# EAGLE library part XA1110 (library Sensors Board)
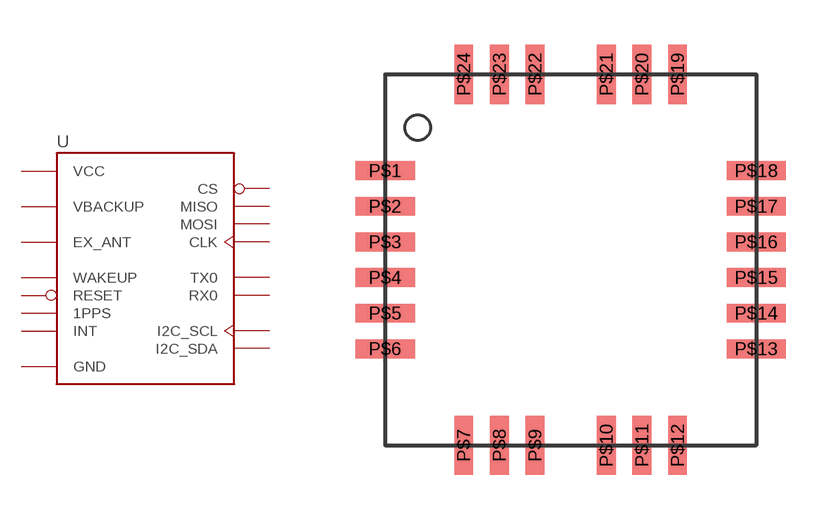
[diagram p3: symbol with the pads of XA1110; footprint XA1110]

Designator prefix -

## XA1110  [XA1110]
P$1  GND  sup
P$2  EX_ANT  in
P$3  GND  sup
P$4  GND  sup
P$5  GND  sup
P$6  GND  sup
P$7  VCC  sup
P$8  VBACKUP  sup
P$9  GND  sup
P$10  GND  sup
P$11  GND  sup
P$12  WAKEUP
P$13  I2C_SDA
P$14  I2C_SCL  in
P$15  MISO  out
P$16  INT  out
P$17  MOSI  in
P$18  CLK  in
P$19  TX0  out
P$20  RX0  in
P$21  1PPS  out
P$22  RESET  in
P$23  CS  in
P$24  GND  sup

## Footprint XA1110 (pad centres in mm)
smd 2 x 0.635: P$1 -6.25,3; P$2 -6.25,1.8; P$3 -6.25,0.6; P$4 -6.25,-0.6; P$5 -6.25,-1.8; P$6 -6.25,-3; P$13 6.25,-3; P$14 6.25,-1.8; P$15 6.25,-0.6; P$16 6.25,0.6; P$17 6.25,1.8; P$18 6.25,3
smd 0.635 x 2: P$7 -3.6,-6.25; P$8 -2.4,-6.25; P$9 -1.2,-6.25; P$10 1.2,-6.25; P$11 2.4,-6.25; P$12 3.6,-6.25; P$19 3.6,6.25; P$20 2.4,6.25; P$21 1.2,6.25; P$22 -1.2,6.25; P$23 -2.4,6.25; P$24 -3.6,6.25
